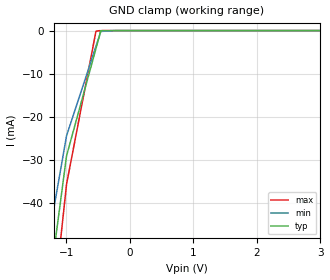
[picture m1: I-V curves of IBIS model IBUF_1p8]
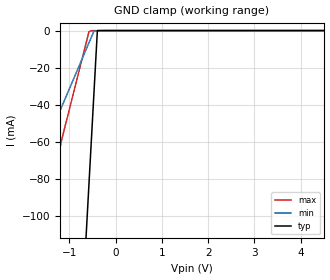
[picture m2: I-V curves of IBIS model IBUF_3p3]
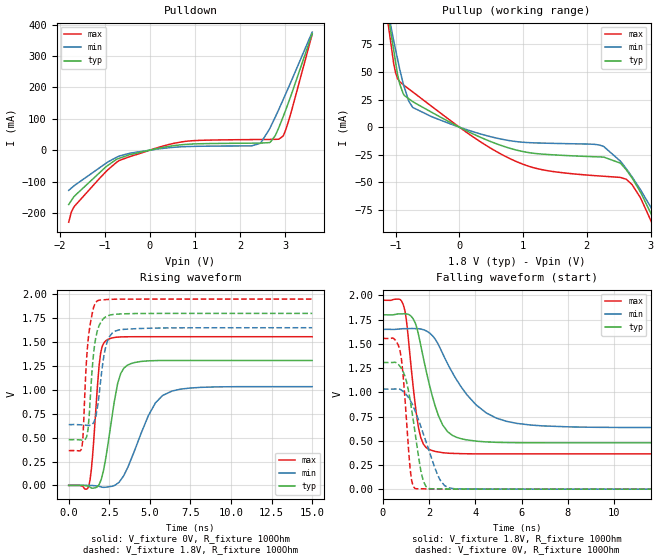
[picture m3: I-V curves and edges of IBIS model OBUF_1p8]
|Texas Instruments Incorporated
| Industry's Lowest-Power,12-Bit, 1-MSPS, SAR ADC
| in Industry's Smallest Package
| Marketing part#   Digital Voltage Range   Package-type   #pins
| ADS7C00S   1.65V - 3.6V   QFN   8
[IBIS Ver]   4.1
[File name]   ads7c00s.ibs
[File Rev]   1.0
[Date]   01/13/2014
[Source]
| Texas Instruments Incorporated.
| 12500 TI Blvd
| Dallas, TX -75243
[Notes]   Revision History:
| Rev 1.0: 01/13/2014
| - Initial version of the model
| - Model generated from simulations in TISPICE
| - C_comp although listed in numerical order of value are
|   obtained from varying PVT conditions. For PVT conditions for
|   each specific value refer the buffer description under
|   respective [Model]. IBIS model user is responsible for using
|   appropriate C_comp to simulate for Signal Integrity.
| - Warnings regarding Non-monotonicity of various models were result
|   of simulaions and have been reviewd and considered minor
|   and can be ignored.
| - Model names with a trailing _1p8 contains the model for
|   1.8V operation.Model names with a trailing _3p3 contains the model
|   for 3.3V operation.
[Disclaimer]
| This model is designed as an aid for customers of Texas Instruments.
| TI and its licensors and suppliers make no warranties, either expressed
| or implied, with respect to this  model, including the warranties of
| merchantability or fitness for a particular purpose. The model is
| provided solely on an "as is" basis. The entire risk as to its quality
| and performance is with the customer.
[Copyright]
 (C) Copyright 2014 Texas Instruments Incorporated.All rights reserved.
|   Device
[Component]   TPS51219
[Manufacturer]   TI
[Package]
| variable   typ   min   max
R_pkg   0.01   0.008   0.12
L_pkg   1.0nH   0.8nH   1.2nH
C_pkg   0.2pF   0.16pF   0.24pF
[Pin]  signal_name   model_name   R_pin   L_pin   C_pin
1   CSB   IBUF   NA   NA   NA
2   SDO   OBUF   NA   NA   NA
3   SCLK   IBUF   NA   NA   NA
4   DVDD   POWER   NA   NA   NA
5   GND   GND   NA   NA   NA
6   AVDD   POWER   NA   NA   NA
7   AINP   NC   NA   NA   NA
8   AINM   NC   NA   NA   NA
|   Model Selectors
[Model Selector]  IBUF
IBUF_3p3  input buffer at 3.3V operation
IBUF_1p8  input buffer at 1.8V operation
[Model Selector]  OBUF
OBUF_3p3  input buffer at 3.3V operation
OBUF_1p8  input buffer at 1.8V operation
| Models and submodels in the file (4): IBUF_1p8 (Input), IBUF_3p3 (Input), OBUF_1p8 (Output), OBUF_3p3 (Output)
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|   Model
[Model]   IBUF_1p8
Model_type   Input
Vinl = 0.63
Vinh = 1.17
|   typ   min   max
C_comp   1.990pF   1.803pF   2.168pF
[Voltage Range]   1.8   1.65   1.95
[Temperature Range]   27   125   -40
[Power Clamp Reference]   1.8   1.65   1.95
[GND Clamp Reference]   0   0   0
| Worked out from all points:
|   GND clamp passes 1 mA (typ) near -0.47 V on its own axis
[GND Clamp]
|   Voltage   I(typ)   I(min)   I(max)
-1.8V     -147.7mA   -99.44mA   -215.5mA
-1.438V   -78.67mA   -61.91mA   -97.03mA
-995.4mV  -29.14mA   -24.49mA   -35.76mA
-532.5mV  -4.201mA   -3.661mA   -173.8uA
-455.4mV  -46.68uA   -193uA     -14.23uA
-212.4mV  -2.827nA   -568.5nA   0A
3.6V      0A         0A         0A
[POWER Clamp]
|   Voltage   I(typ)   I(min)   I(max)
-1.8V     0A         0A         0A
-1.789V   0A         0A         0A
-369mV    0A         0A         0A
3.6V      0A         0A         0A
|   Model
[Model]   IBUF_3p3
Model_type   Input
Vinl = 1.155
Vinh = 2.145
|   typ   min   max
C_comp   1.990pF   1.803pF   2.168pF
[Voltage Range]   3.3   3   3.6
[Temperature Range]   27   125   -40
[Power Clamp Reference]   3.3   3   3.6
[GND Clamp Reference]   0   0   0
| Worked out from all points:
|   GND clamp passes 1 mA (typ) near -0.40 V on its own axis
[GND Clamp]
|   Voltage   I(typ)   I(min)   I(max)
-3.3V     -1.546A    -1.399A    -1.656A
-2.637V   -1.021A    -758.9mA   -1.004A
-1.825V   -651.2mA   -104.5mA   -235.8mA
-1.597V   -547.5mA   -76.71mA   -127.2mA
-1.518V   -511.4mA   -69.27mA   -108.8mA
-1.28V    -403.2mA   -47.79mA   -74.48mA
-1.181V   -358.1mA   -41.99mA   -60.37mA
-577.4mV  -82.93mA   -6.622mA   -583uA
-567.6mV  -78.48mA   -6.049mA   -455.2uA
-468.6mV  -33.38mA   -251.2uA   -22.72uA
-395.3mV  -8.029uA   -170.8uA   -2.084uA
6.6V      0A         0A         0A
[POWER Clamp]
|   Voltage   I(typ)   I(min)   I(max)
-3.3V     0A         0A         0A
-3.28V    0A         0A         0A
-448.8mV  0A         0A         0A
6.6V      0A         0A         0A
|   Model
[Model]   OBUF_1p8
Model_type   Output
Polarity   Non-Inverting
Vmeas = 0.9
Vref = 0
Cref = 1pF
Rref = 10000
|   typ   min   max
C_comp   2.314pF   1.935pF   2.523pF
[Voltage Range]   1.8   1.65   1.95
[Temperature Range]   27   125   -40
[Pullup Reference]   1.8   1.65   1.95
[Pulldown Reference]   0   0   0
[Power Clamp Reference]   1.8   1.65   1.95
[GND Clamp Reference]   0   0   0
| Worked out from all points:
|   slope of the pulldown table from 0 to 0.27 V, typ, clamps not added: 33.1 ohm
|   slope of the pullup table from 0 to 0.27 V, typ, clamps not added: 35.7 ohm
|   falling waveform, V_fixture 1.8V, R_fixture 100Ohm: 20-80 % time 838ps typ, 1.7ns min, 441ps max; typ from 1.8 V to 0.478 V
|   rising waveform, V_fixture 0V, R_fixture 100Ohm: 20-80 % time 732ps typ, 1.54ns min, 396ps max; typ from 0 V to 1.31 V
|   rising waveform, V_fixture 1.8V, R_fixture 100Ohm: 20-80 % time 391ps typ, 486ps min, 350ps max; typ from 0.478 V to 1.8 V
|   falling waveform, V_fixture 0V, R_fixture 100Ohm: 20-80 % time 511ps typ, 909ps min, 296ps max; typ from 1.31 V to 0 V
[Pulldown]
|   Voltage   I(typ)   I(min)   I(max)
-1.8V     -173.4mA   -128.1mA   -229.7mA
-1.743V   -161mA     -121.2mA   -198.1mA
-1.66V    -144.7mA   -111.3mA   -176.8mA
-984.6mV  -54.49mA   -43.03mA   -70.17mA
-676.8mV  -25.77mA   -18.73mA   -32.83mA
711mV     17.31mA    10.75mA    26.38mA
2.455V    22.44mA    22mA       33.92mA
2.671V    25.28mA    72.32mA    34.18mA
2.779V    45.8mA     104.7mA    34.38mA
2.957V    106.9mA    161.3mA    45.35mA
3.146V    180.7mA    223.5mA    127.3mA
3.6V      371mA      376.4mA    369.5mA
[Pullup]
|   Voltage   I(typ)   I(min)   I(max)
-1.8V     373.3mA    326.1mA    457.3mA
-1.12V    102.4mA    105.3mA    94.79mA
-1.028V   69.08mA    77.63mA    56.95mA
-968.4mV  47.5mA     61.49mA    43.96mA
-882mV    30.48mA    39.64mA    38.47mA
-730.8mV  23.03mA    17.84mA    31.83mA
84.6mV    -2.469mA   -1.685mA   -3.535mA
873mV     -20.41mA   -12.91mA   -30.59mA
2.255V    -27.08mA   -17.33mA   -44.39mA
2.617V    -38.49mA   -37.49mA   -47.11mA
3.157V    -96.25mA   -87.51mA   -104.1mA
3.6V      -167mA     -168.8mA   -172.6mA
[Ramp]
R_load = 100
|   typ   min   max
dV/dt_r   0.784406/7.32265e-10   0.61994/1.53788e-09   0.933554/3.95806e-10
dV/dt_f   0.792922/8.3829e-10   0.608415/1.704e-09   0.95148/4.41219e-10
[Falling Waveform]
V_fixture = 1.8V
V_fixture_min = 1.65V
V_fixture_max = 1.95V
R_fixture = 100Ohm
C_fixture = 0F
|   Time   V(typ)   V(min)   V(max)
0s        1.8V       1.65V      1.95V
923ps     1.81V      1.657V     1.874V
1.273ns   1.772V     1.658V     1.148V
1.543ns   1.595V     1.656V     636.3mV
2.055ns   1.04V      1.605V     405.5mV
2.587ns   663.2mV    1.401V     377mV
3.016ns   554.1mV    1.2V       369.3mV
4.035ns   495.9mV    869.4mV    364.7mV
5.347ns   481.2mV    700.2mV    364.2mV
15ns      478.5mV    636mV      364.2mV
[Rising Waveform]
V_fixture = 0V
V_fixture_min = 0V
V_fixture_max = 0V
R_fixture = 100Ohm
C_fixture = 0F
|   Time   V(typ)   V(min)   V(max)
0s        258.6nV    -86.47nV   2.136nV
1.245ns   -10.97mV   35.41uV    -1.931mV
1.467ns   -28.92mV   -1.518mV   301.3mV
1.968ns   47.81mV    -13.82mV   1.384V
2.392ns   400.2mV    -15.94mV   1.526V
3.016ns   1.067V     22.25mV    1.552V
3.814ns   1.273V     260.9mV    1.556V
5.347ns   1.306V     864.8mV    1.556V
6.376ns   1.308V     988.4mV    1.556V
15ns      1.307V     1.033V     1.556V
[Rising Waveform]
V_fixture = 1.8V
V_fixture_min = 1.65V
V_fixture_max = 1.95V
R_fixture = 100Ohm
C_fixture = 0F
|   Time   V(typ)   V(min)   V(max)
0s        478.4mV    636.1mV    364.1mV
806.8ps   474.7mV    633.5mV    392mV
868.3ps   473.7mV    633mV      471.2mV
1.05ns    490.5mV    630mV      1.168V
1.188ns   582.4mV    627.8mV    1.507V
1.497ns   1.318V     648.5mV    1.836V
1.755ns   1.612V     801mV      1.931V
2.274ns   1.764V     1.445V     1.944V
2.862ns   1.791V     1.614V     1.949V
15ns      1.8V       1.65V      1.95V
[Falling Waveform]
|Gnd
V_fixture = 0V
V_fixture_min = 0V
V_fixture_max = 0V
R_fixture = 100Ohm
C_fixture = 0F
|   Time   V(typ)   V(min)   V(max)
0s        1.307V     1.033V     1.556V
756.6ps   1.263V     1.029V     1.415V
868.3ps   1.218V     1.011V     1.201V
1.188ns   910mV      915.7mV    195mV
1.396ns   582.1mV    808.5mV    6.463mV
1.662ns   167.9mV    634.3mV    4.245mV
1.873ns   25.57mV    486mV      2.83mV
2.444ns   3.33mV     109.7mV    1.056mV
2.862ns   1.878mV    12.82mV    616.2uV
15ns      -317.8nV   -1.092uV   100.1nV
